| Texas Instruments Incorporated
| Low-Noise Clock Jitter Cleaner with Dual Loop PLLs
| Marketing part#   Voltage Range   Package-type   #pins/pkg drawing
| LMK04808   3.15V - 3.45V   LLP   64-pin SQ
[IBIS Ver]   4.1
[File name]   lmk04808.ibs
[File Rev]   1.6
[Date]   11/12/2015
[Source]   Model built from spectre simulations at:
   Texas Instruments Incorporated.
   Analog-eLab, HPA
   12500 TI Blvd
   Dallas, TX -75243
   For Support e-mail: elab_ibis@list.ti.com
[Notes]   Revision History
   Rev 1.0: 5/07/2012
   -PullUp and Pulldown non-monotonic for LVPECL models
   -LVPECL simulation recommendation:
   It is recommended that a small (1nF or less) AC coupling cap
   be used. Larger values will result in long settling times
   - C_comp although listed in numberical order of value are obtained from varying PVT conditions.
   For PVT conditions for each specific value, refer to the buffer description under repective [Model].
   IBIS model user is responsible for using appropriate C_comp to simulate for Signal Integrity.
   Rev 1.1: 5/08/2012
   -Update OSCIN and CLKIN input buffer models
   Rev 1.2: 5/22/2012
   -Update LVDS model
   Rev 1.3: 2/05/2013
   -Update name of CLKIN to CLKIN_BJT to differentiate this mode from CMOS mode.
   Rev 1.4: 11/11/2013
   - Update UWIRE_DIN model
   - Add SYNC model
   - Add STATUS model
   - Combined Pullup and Pulldown non-monotonic for STATUS model
   Rev 1.5: 10/27/2014
   - Correct Package model assignment, add package pin data
   - Remove Rising and Falling VT data from LVPECL outputs to better match bench
   Rev 1.6: 11/12/2015
   - Correct vinh/vinl in UWIRE_DIN model
[Disclaimer]  This model is designed as an aid for customers of Texas Instruments
 TI and its licensors and suppliers make no warranties, either expressed
 or implied, with respect to this  model, including the warranties of
 merchantability or fitness for a particular purpose.
 The model is provided solely on an "as is" basis. The entire risk as to
 its quality and performance is with the customer.
[Copyright] (C)Copyright 2013 Texas Instruments Incorporated.
   All rights reserved.
[Component]   LMK04808BISQ
[Manufacturer]  Texas Instruments Incorporated
[Package]   |64-pin LLP SQ package
|   typ   min   max
R_pkg   0.8083   0.2082   1.1685
L_pkg   1.9144n   0.9780n   2.5932n
C_pkg   0.2940p   0.2235p   0.3750p
[Pin]   signal_name   model_name   R_pin   L_pin   C_pin
1   CLKOUT0   TRI_MODE_OUT   1.0479   2.2614n   0.3102p
2   CLKOUT0*   TRI_MODE_OUT   0.9280   2.0696n   0.2990p
3   CLKOUT1*   TRI_MODE_OUT   0.9076   1.9169n   0.2964p
4   CLKOUT1   TRI_MODE_OUT   0.7860   1.7984n   0.2662p
5   BIAS   NC   0.7397   1.6454n   0.2566p
6   SYNC   SYNC   0.6580   1.6443n   0.2235p
7   NC   NC   0.8083   1.9144n   0.2940p
8   NC   NC   0.2082   0.9780n   0.3750p
9   NC   NC   0.8083   1.9144n   0.2940p
10   VCC1   POWER   0.6675   1.4601n   0.2362p
11   LDOBYP1   NC   0.6633   1.6138n   0.2394p
12   LDOBYP2   NC   0.7420   1.6705n   0.2565p
13   CLKOUT2   TRI_MODE_OUT   0.7864   1.7943n   0.2681p
14   CLKOUT2*   TRI_MODE_OUT   0.9061   1.9343n   0.2945p
15   CLKOUT3*   TRI_MODE_OUT   0.9417   2.0541n   0.3033p
16   CLKOUT3   TRI_MODE_OUT   1.0450   2.2863n   0.3073p
17   VCC2   POWER   0.5439   1.9925n   0.3083p
18   VCC3   POWER   0.6208   1.8410n   0.3548p
19   CLKOUT4   TRI_MODE_OUT   1.0434   2.1334n   0.3225p
20   CLKOUT4*   TRI_MODE_OUT   0.9542   2.0383n   0.3001p
21   CLKOUT5*   TRI_MODE_OUT   0.9298   1.9770n   0.2928p
22   CLKOUT5   TRI_MODE_OUT   0.8633   1.9431n   0.2749p
23   GND   GND   0.4944   1.5389n   0.3209p
24   VCC4   POWER   0.4513   1.5949n   0.3085p
25   CLKIN1   CLKIN   0.7761   2.0010n   0.2589p
26   CLKIN1*   CLKIN   0.7888   2.0399n   0.2595p
27   STATUS_HOLDOVER STATUS_SEL   0.8372   2.0300n   0.2601p
28   CLKIN0   CLKIN   0.8778   1.9970n   0.2766p
29   CLKIN0*   CLKIN   0.9549   2.0555n   0.2956p
30   VCC5   POWER   0.6176   1.6773n   0.3714p
31   OSCOUT1   OSCOUT   0.9873   2.2321n   0.3058p
32   OSCOUT1*   OSCOUT   1.0155   2.5932n   0.2924p
33   STATUS_LD   STATUS_SEL   1.0562   2.4339n   0.2970p
34   CPOUT1   NC   1.0279   2.1272n   0.3171p
35   VCC6   POWER   0.5777   1.6206n   0.3720p
36   OSCIN   OSCIN   0.9257   2.0512n   0.2910p
37   OSCIN*   OSCIN   0.8488   1.9597n   0.2725p
38   VCC7   POWER   0.5091   1.4436n   0.3284p
39   OSCOUT0   OSCOUT   0.7887   1.7936n   0.2637p
40   OSCOUT0*   OSCOUT   0.7794   1.6957n   0.2636p
41   VCC8   POWER   0.4498   1.2960n   0.3176p
42   CPOUT2   NC   0.7591   1.7186n   0.2560p
43   VCC9   POWER   0.7654   1.7601n   0.2533p
44   LEUWIRE   UWIRE_DIN   0.7788   1.8176n   0.2606p
45   CLKUWIRE   UWIRE_DIN   0.8019   2.0498n   0.2623p
46   DATAUWIRE   UWIRE_DIN   0.8551   2.1817n   0.2776p
47   VCC10   POWER   0.5509   1.8732n   0.3295p
48   CLKOUT6   TRI_MODE_OUT   1.1185   2.3922n   0.3166p
49   CLKOUT6*   TRI_MODE_OUT   1.1228   2.4432n   0.3171p
50   CLKOUT7*   TRI_MODE_OUT   1.1685   2.3406n   0.3461p
51   CLKOUT7   TRI_MODE_OUT   1.0374   2.2717n   0.3156p
52   VCC11   POWER   0.6154   1.6880n   0.3737p
53   CLKOUT8   TRI_MODE_OUT   0.9641   2.0390n   0.2986p
54   CLKOUT8*   TRI_MODE_OUT   0.8853   1.9486n   0.2812p
55   CLKOUT9*   TRI_MODE_OUT   0.8702   1.8830n   0.2797p
56   CLKOUT9   TRI_MODE_OUT   0.8238   1.8596n   0.2666p
57   VCC12   POWER   0.4907   1.4278n   0.3203p
58   CLKOUT10   TRI_MODE_OUT   0.8223   1.8286n   0.2691p
59   CLKOUT10*   TRI_MODE_OUT   0.8277   1.8868n   0.2674p
60   CLKOUT11*   TRI_MODE_OUT   0.8684   1.8586n   0.2799p
61   CLKOUT11   TRI_MODE_OUT   0.9011   2.0080n   0.2815p
62   STATUS_CLKIN0   STATUS_SEL   0.9334   2.1446n   0.2820p
63   STATUS_CLKIN1   STATUS_SEL   0.8912   2.3255n   0.2704p
64   VCC13   POWER   0.5148   1.7149n   0.3615p
65   DAP   GND   0.0135   0.0533n   11.945p
[Package Model] llp64_lmk04808_base
[Diff pin]  inv_pin  vdiff  tdelay_typ  tdelay_min  tdelay_max
 1   2   0.0   0.0s   0.0s   0.0s
 4   3   0.0   0.0s   0.0s   0.0s
13   14   0.0   0.0s   0.0s   0.0s
16   15   0.0   0.0s   0.0s   0.0s
19   20   0.0   0.0s   0.0s   0.0s
22   21   0.0   0.0s   0.0s   0.0s
25   26   0.0   0.0s   0.0s   0.0s
31   32   0.0   0.0s   0.0s   0.0s
36   37   0.0   0.0s   0.0s   0.0s
39   40   0.0   0.0s   0.0s   0.0s
48   49   0.0   0.0s   0.0s   0.0s
51   50   0.0   0.0s   0.0s   0.0s
53   54   0.0   0.0s   0.0s   0.0s
56   55   0.0   0.0s   0.0s   0.0s
58   59   0.0   0.0s   0.0s   0.0s
61   60   0.0   0.0s   0.0s   0.0s
[Model Selector] TRI_MODE_OUT
LVPECL0P7   LVPECL 0.7V OUTPUT
LVPECL1P2   LVPECL 1.2V OUTPUT
LVPECL1P6   LVPECL 1.6V OUTPUT
LVPECL2P0   LVPECL 2.0V OUTPUT
LVDS   LVDS OUTPUT
LVCMOS   LVCMOS OUTPUT
[Model Selector] OSCOUT
LVPECL0P7   LVPECL 0.7V OUTPUT
LVPECL1P2   LVPECL 1.2V OUTPUT
LVPECL1P6   LVPECL 1.6V OUTPUT
LVPECL2P0   LVPECL 2.0V OUTPUT
[Model Selector] CLKIN
CLKIN_BJT   CLKIN Bipolar Input
|CLKIN_CMOS   CLKIN CMOS Input
[Model Selector] STATUS_SEL
STATUS   SWITCHING OUTPUT
TERM_PU   TERMINATOR, WEAK PULL UP
TERM_PD   TERMINATOR, WEAK PULL DOWN
[Define Package Model]  llp64_lmk04808_base
[Manufacturer]  Unknown
[OEM]  Unknown
[Description]  Package Model at 5GHz
[Number Of Pins]  63
[Pin Numbers]
65   | 65 = DAP
1   | 1 = L1
2   | 2 = L2
3   | 3 = L3
4   | 4 = L4
5   | 5 = L5
6   | 6 = L6
8   | 8 = L8
10   | 10 = L10
11   | 11 = L11
12   | 12 = L12
13   | 13 = L13
14   | 14 = L14
15   | 15 = L15
16   | 16 = L16
17   | 17 = L17
18   | 18 = L18
19   | 19 = L19
20   | 20 = L20
21   | 21 = L21
22   | 22 = L22
23   | 23 = L23
24   | 24 = L24
25   | 25 = L25
26   | 26 = L26
27   | 27 = L27
28   | 28 = L28
29   | 29 = L29
30   | 30 = L30
31   | 31 = L31
32   | 32 = L32
33   | 33 = L33
34   | 34 = L34
35   | 35 = L35
36   | 36 = L36
37   | 37 = L37
38   | 38 = L38
39   | 39 = L39
40   | 40 = L40
41   | 41 = L41
42   | 42 = L42
43   | 43 = L43
44   | 44 = L44
45   | 45 = L45
46   | 46 = L46
47   | 47 = L47
48   | 48 = L48
49   | 49 = L49
50   | 50 = L50
51   | 51 = L51
52   | 52 = L52
53   | 53 = L53
54   | 54 = L54
55   | 55 = L55
56   | 56 = L56
57   | 57 = L57
58   | 58 = L58
59   | 59 = L59
60   | 60 = L60
61   | 61 = L61
62   | 62 = L62
63   | 63 = L63
64   | 64 = L64
[Model Data]
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[End Model Data]
[End Package Model]
| Models and submodels in the file (13): UWIRE_DIN (Input), SYNC (Input), STATUS (3-state), TERM_PU (Terminator), TERM_PD (Terminator), CLKIN_BJT (Input), OSCIN (Input), LVCMOS (Output), LVDS (Output), LVPECL0P7 (Output), LVPECL1P2 (Output), LVPECL1P6 (Output), LVPECL2P0 (Output)
